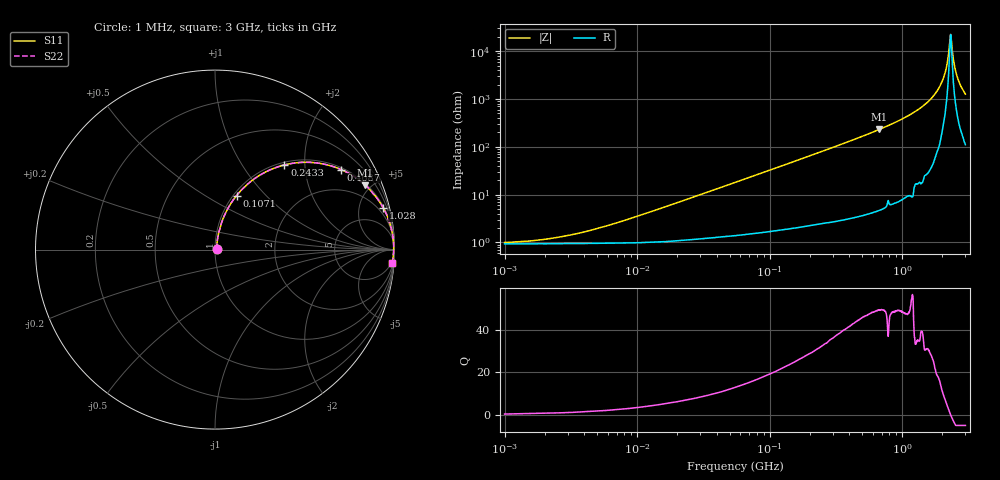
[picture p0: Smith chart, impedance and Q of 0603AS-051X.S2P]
!s-Parameter Generated by FASTRON Sdn. Bhd.
!FASTRON P/N : 0603AS-051X
!Keysight Technologies: E4991B_MY54100416_A.01.15
!Date created: Wed Oct 04 11:45:39 2023
!Version  : Rev01 Wed Oct 04 11:45:39 2023
!Data & Calibration Information:
!Freq	S11	S21	S12	S22
!PortZ  Port1:50+j0  Port2:50+j0
!When reading reference impedance value at option line is always used.
! Remarks : This data is being provided solely for informational purposes.
# Hz S dB R 50
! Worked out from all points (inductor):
!   1601 points, 1 MHz to 3 GHz, reference 50 ohm
!   read as one part in series: L = 53.8 nH near 8.686 MHz
!   highest Q = 49.4 at 671.9 MHz (marker M1), where L = 54.9 nH
!   self-resonance near 2.313 GHz
!   S11 on the Smith chart (normalised r, x): 1 MHz: 1.02, +0.01; 107.1 MHz: 1.03, +0.70; 243.3 MHz: 1.05, +1.57; 468.7 MHz: 1.07, +3.10; 1.028 GHz: 1.17, +7.99; 3 GHz: 3, -25
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1000000  -40.10 19.9  -0.08 -0.2  -0.08 -0.2  -40.10 19.9
3804036  -35.94 53.0  -0.08 -0.7  -0.08 -0.7  -35.94 53.0
1.447069e7  -26.16 75.4  -0.10 -2.8  -0.10 -2.8  -26.16 75.4
5.477226e7  -15.14 75.5  -0.25 -10.0  -0.25 -10.0  -15.14 75.5
1.070951e8  -9.80 68.3  -0.63 -18.9  -0.63 -18.9  -9.80 68.3
2.083556e8  -5.19 54.7  -1.76 -33.4  -1.76 -33.4  -5.19 54.7
2.433181e8  -4.30 50.7  -2.23 -37.5  -2.23 -37.5  -4.30 50.7
4.686663e8  -1.60 32.4  -5.41 -56.3  -5.41 -56.3  -1.60 32.4
6.719458e8  -0.81 23.2  -8.10 -65.7  -8.10 -65.7  -0.81 23.2
7.925923e8  -0.58 19.4  -9.57 -69.2  -9.57 -69.2  -0.58 19.4
1.02815e9  -0.31 14.0  -12.34 -74.8  -12.34 -74.8  -0.31 14.0
1.466741e9  -0.11 7.5  -17.63 -80.6  -17.63 -80.6  -0.11 7.5
1.837163e9  -0.05 3.8  -23.47 -83.1  -23.47 -83.1  -0.05 3.8
2.081985e9  -0.04 1.8  -30.00 -81.1  -30.00 -81.1  -0.04 1.8
2.167021e9  -0.04 1.1  -33.82 -77.6  -33.82 -77.6  -0.04 1.1
2.266846e9  -0.04 0.4  -41.84 -58.3  -41.84 -58.3  -0.04 0.4
2.312676e9  -0.04 0.1  -46.86 -14.8  -46.86 -14.8  -0.04 0.1
2.383164e9  -0.04 -0.4  -41.10 58.2  -41.10 58.2  -0.04 -0.4
2.492946e9  -0.05 -1.2  -33.42 75.3  -33.42 75.3  -0.05 -1.2
2.607784e9  -0.05 -2.0  -29.24 79.1  -29.24 79.1  -0.05 -2.0
2.797026e9  -0.07 -3.2  -25.07 80.3  -25.07 80.3  -0.07 -3.2
3e9  -0.09 -4.4  -22.18 80.5  -22.18 80.5  -0.09 -4.4
